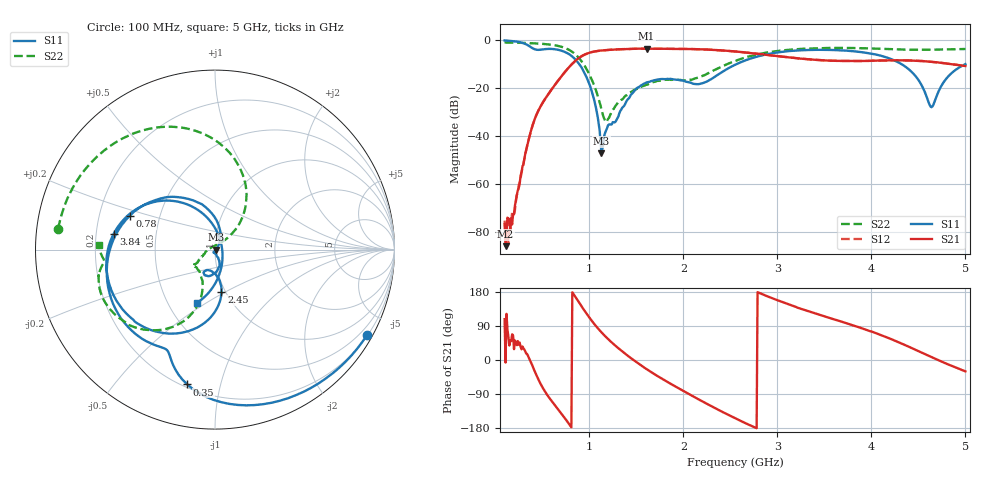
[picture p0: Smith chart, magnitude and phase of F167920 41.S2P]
!  2-Port S-parameters saved by WinCal
! VAR MeasName=S-Parameters (CALIBRATED_DATA) read from VNA (N5242A)
! VAR MeasDate=2016-11-22 9:57:28
! VAR NAME=F167920 41
! VAR FILENAME=F167920 41.S2P
! VAR DATE=2016-11-22 9:57:28
! VAR PHYS_PORTS=1,2
# Hz S DB R 50
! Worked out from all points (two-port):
!   491 points, 100 MHz to 5 GHz, reference 50 ohm
!   highest |S21| = -3.65 dB at 1.61 GHz (marker M1); lowest = -85.9 dB at 110 MHz (marker M2)
!   |S21| within 3 dB of the highest: 925.2 MHz to 2.973 GHz (2.048 GHz wide, 105 % of centre)
!   lowest |S11| = -47.3 dB at 1.13 GHz (marker M3), VSWR 1.01, Z = 50.4 - j0.101 ohm
!   |S11| at or under -10 dB: 891.6 MHz to 2.571 GHz (1.68 GHz wide, 97 % of centre); 4.316 GHz to end of sweep
!   |S22| runs from -34.2 to -1.1 dB; largest |S21 - S12| = 0.0015
!   S11 on the Smith chart (normalised r, x): 100 MHz: 0.22, -3.82; 350 MHz: 0.22, -0.79; 780 MHz: 0.33, +0.17; 2.45 GHz: 0.96, -0.48; 3.84 GHz: 0.27, +0.07; 5 GHz: 0.70, -0.46
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1e8  -0.25 -29.3  -76.66 107.8  -75.26 104.5  -1.10 172.4
1.1e8  -0.28 -32.1  -85.90 -6.8  -79.84 134.7  -1.10 171.6
1.8e8  -0.51 -52.2  -76.86 67.8  -71.84 40.5  -1.15 166.3
3.5e8  -2.31 -101.6  -42.60 10.2  -42.45 10.0  -1.34 152.2
4.8e8  -4.11 -119.9  -27.88 -61.7  -27.86 -61.6  -1.61 139.4
7.8e8  -5.83 158.4  -11.61 -167.0  -11.60 -167.0  -4.05 92.5
9.2e8  -11.59 106.2  -6.77 141.4  -6.76 141.4  -9.03 60.2
1.04e9  -23.23 64.4  -4.98 99.2  -4.98 99.2  -17.75 43.4
1.13e9  -47.30 -13.4  -4.43 73.0  -4.43 73.1  -28.99 58.8
1.19e9  -36.71 -117.5  -4.21 57.7  -4.20 57.7  -33.70 133.6
1.61e9  -17.71 -89.5  -3.65 -24.1  -3.65 -24.1  -18.70 -145.3
1.74e9  -16.43 -102.3  -3.71 -44.4  -3.70 -44.4  -17.08 -144.3
2.08e9  -17.83 -113.7  -3.80 -92.4  -3.80 -92.4  -16.65 -128.0
2.45e9  -12.49 -81.2  -4.50 -141.2  -4.50 -141.2  -10.40 -106.7
2.55e9  -10.39 -85.7  -4.82 -153.5  -4.82 -153.5  -8.80 -109.0
3.37e9  -4.18 -152.0  -8.22 125.3  -8.21 125.3  -3.55 -147.4
3.84e9  -4.87 171.2  -8.82 88.6  -8.82 88.5  -3.42 -163.6
4.19e9  -7.70 139.0  -8.55 57.3  -8.56 57.3  -3.84 -171.0
4.46e9  -14.64 104.2  -8.65 28.0  -8.66 28.1  -4.13 -173.8
4.64e9  -28.03 6.1  -9.13 7.6  -9.14 7.7  -4.10 -175.3
4.8e9  -16.01 -84.0  -9.84 -9.9  -9.83 -9.8  -3.95 -177.7
5e9  -10.11 -108.6  -10.92 -30.0  -10.90 -29.9  -3.81 177.7
